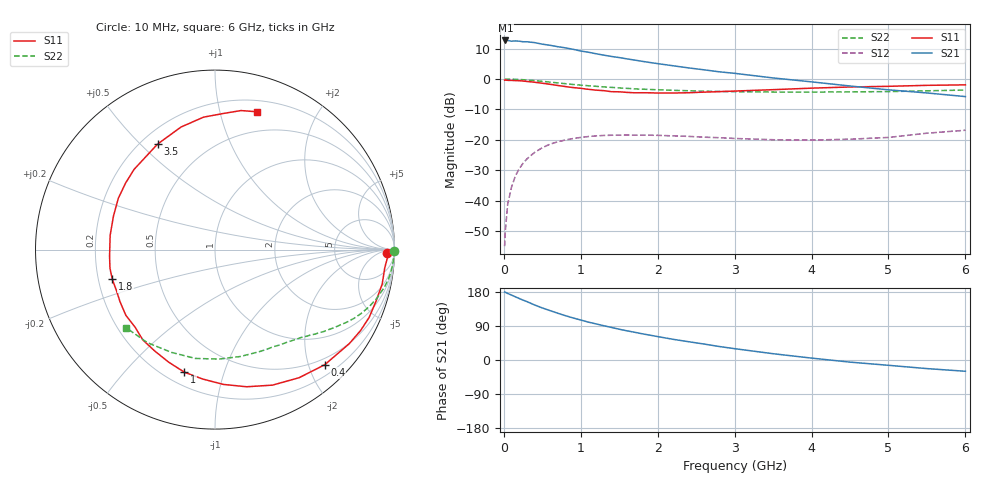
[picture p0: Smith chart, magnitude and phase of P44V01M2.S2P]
! SIEMENS Small Signal Semiconductors
! BFP182
! Si NPN RF Bipolar Junction Transistor in SOT143
! VCE = 4 V  IC = 1.2 mA
! Common Emitter S-Parameters:  March  1996
# GHz  S  MA  R  50
!  f  S11  S21  S12  S22
! GHz  MAG  ANG  MAG  ANG  MAG  ANG  MAG  ANG
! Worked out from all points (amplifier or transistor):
!   36 points, 10 MHz to 6 GHz, reference 50 ohm
!   highest |S21| = 12.7 dB at 20 MHz (marker M1)
!   |S21| within 3 dB of that: start of sweep to 916.8 MHz
!   unconditionally stable (mu >= 1): 2.548 GHz to end of sweep
!   at 250 MHz: K = 0.11, MSG = 20.0 dB, |S12| = -27.7 dB
!   at 1.4 GHz: K = 0.56, MSG = 12.9 dB, |S12| = -18.5 dB
!   at 6 GHz: K = 1.06, MAG = 4.0 dB, |S12| = -16.8 dB
!   S11 on the Smith chart (normalised r, x): 10 MHz: 39, -16; 400 MHz: 0.38, -2.28; 1 GHz: 0.27, -0.74; 1.8 GHz: 0.26, -0.13; 3.5 GHz: 0.26, +0.56; 6 GHz: 0.30, +1.31
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0.01  0.9572 -1.0  4.208 179.5  0.0018 91.3  0.998 -0.4
0.02  0.9632 -2.3  4.303 178.8  0.0033 92.6  0.9908 -0.8
0.05  0.9513 -6.1  4.3 175.6  0.0088 88.0  0.9972 -2.2
0.1  0.9511 -11.6  4.186 171.3  0.0168 81.9  0.994 -4.4
0.15  0.9423 -17.7  4.228 166.8  0.0256 78.4  0.9887 -6.7
0.3  0.9135 -35.0  4.095 154.1  0.0488 68.6  0.9649 -12.8
0.4  0.8861 -46.4  3.966 145.2  0.0624 62.3  0.9421 -16.7
0.5  0.8539 -56.7  3.741 137.4  0.0745 55.7  0.9167 -20.2
0.6  0.8203 -67.0  3.585 130.4  0.0852 50.4  0.8915 -23.3
0.7  0.7843 -77.0  3.398 123.5  0.0932 45.2  0.8651 -26.2
0.8  0.7527 -86.4  3.255 117.0  0.0999 40.3  0.8388 -28.8
1  0.7041 -104.0  2.885 105.5  0.11 32.2  0.795 -33.1
1.1  0.6778 -112.5  2.756 99.9  0.1138 28.8  0.7758 -35.0
1.3  0.6442 -128.6  2.468 90.4  0.1185 22.5  0.7432 -38.5
1.5  0.6171 -143.5  2.254 81.2  0.1196 17.5  0.7144 -41.7
1.8  0.5956 -164.0  1.954 69.1  0.1199 11.9  0.682 -46.2
2.2  0.5895 172.3  1.652 54.6  0.1166 6.0  0.6527 -52.4
2.8  0.6209 143.4  1.315 35.6  0.1089 1.9  0.6259 -62.5
3.5  0.6692 118.6  1.043 16.6  0.1008 2.9  0.6123 -76.5
4.5  0.7408 94.9  0.769 -5.6  0.1028 10.5  0.6162 -100.3
5.5  0.7881 79.4  0.591 -22.7  0.129 17.1  0.641 -126.1
6  0.8029 73.0  0.515 -29.7  0.1442 15.4  0.6596 -138.8
